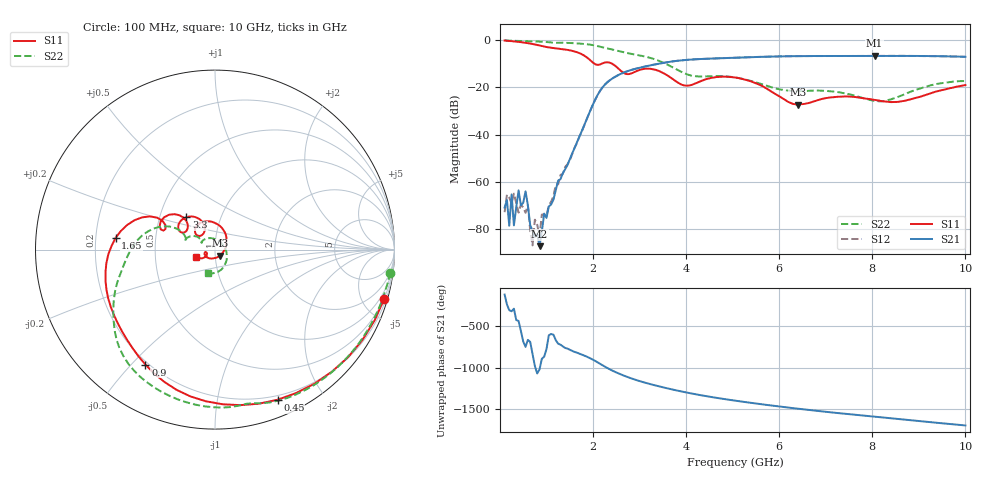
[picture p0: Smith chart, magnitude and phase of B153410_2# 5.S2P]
!  2-Port S-parameters saved by WinCal
! VAR MeasName=S-Parameters (CALIBRATED_DATA) read from VNA (N5245A)
! VAR MeasDate=2016-12-23 9:59:36
! VAR NAME=B153410_2# 5
! VAR FILENAME=B153410_2# 5.S2P
! VAR DATE=2016-12-23 9:59:36
! VAR PHYS_PORTS=1,2
# Hz S DB R 50
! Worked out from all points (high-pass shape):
!   199 points, 100 MHz to 10 GHz, reference 50 ohm
!   highest |S21| = -6.63 dB at 8.05 GHz (marker M1); lowest = -87.2 dB at 850 MHz (marker M2)
!   |S21| within 3 dB of the highest: 3.504 GHz to end of sweep
!   lowest |S11| = -27.3 dB at 6.4 GHz (marker M3), VSWR 1.09, Z = 52.7 - j3.52 ohm
!   |S11| at or under -10 dB: 2.033 GHz to 2.183 GHz (150.1 MHz wide, 7.12 % of centre); 2.411 GHz to end of sweep
!   |S22| runs from -25.9 to -0.1 dB; largest |S21 - S12| = 0.0021
!   S11 on the Smith chart (normalised r, x): 100 MHz: 0.45, -7.02; 450 MHz: 0.16, -1.49; 900 MHz: 0.19, -0.55; 1.65 GHz: 0.28, +0.05; 3.3 GHz: 0.68, +0.26; 10 GHz: 0.81, -0.07
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1e8  -0.15 -16.2  -70.85 -118.1  -72.79 -61.1  -0.14 -7.5
1.5e8  -0.24 -23.9  -67.62 122.7  -65.39 -176.1  -0.18 -10.9
2e8  -0.32 -31.5  -78.55 52.8  -66.65 171.2  -0.22 -14.3
2.5e8  -0.41 -39.0  -65.29 40.1  -69.16 31.1  -0.24 -17.6
3e8  -0.52 -46.3  -78.37 71.1  -64.94 24.0  -0.28 -21.0
4e8  -0.74 -60.5  -63.55 -77.1  -72.98 -45.0  -0.34 -27.6
4.5e8  -0.85 -67.4  -69.91 162.8  -69.70 159.8  -0.37 -30.9
5.5e8  -1.13 -80.7  -63.96 -29.3  -73.08 85.3  -0.42 -37.5
6.5e8  -1.45 -93.5  -78.31 30.7  -80.56 168.1  -0.48 -44.1
8.5e8  -2.28 -116.2  -87.18 58.8  -82.99 -126.7  -0.63 -57.2
9e8  -2.51 -121.2  -80.98 -173.3  -73.82 -159.3  -0.68 -60.5
1.65e9  -5.07 173.3  -43.45 -98.5  -43.68 -97.4  -1.37 -106.9
1.75e9  -5.89 164.3  -38.85 -120.9  -39.08 -121.2  -1.51 -113.5
2.3e9  -9.35 152.6  -17.95 77.5  -17.92 77.5  -3.52 -148.1
3.3e9  -12.36 131.7  -10.39 -129.3  -10.39 -129.3  -7.93 167.1
3.4e9  -12.93 125.1  -10.02 -143.5  -10.00 -143.5  -8.63 162.4
5.05e9  -15.81 103.3  -7.42 41.7  -7.44 41.7  -15.76 154.3
6.4e9  -27.30 -50.5  -6.77 -55.4  -6.78 -55.3  -21.56 153.3
6.7e9  -26.21 -97.5  -6.72 -74.4  -6.73 -74.5  -21.37 151.5
8.05e9  -25.21 -166.2  -6.63 -152.9  -6.64 -152.9  -25.70 61.4
8.35e9  -26.14 -160.6  -6.65 -169.4  -6.64 -169.4  -25.29 17.3
1e10  -19.02 -158.6  -7.06 102.4  -7.06 102.4  -17.30 -106.8
